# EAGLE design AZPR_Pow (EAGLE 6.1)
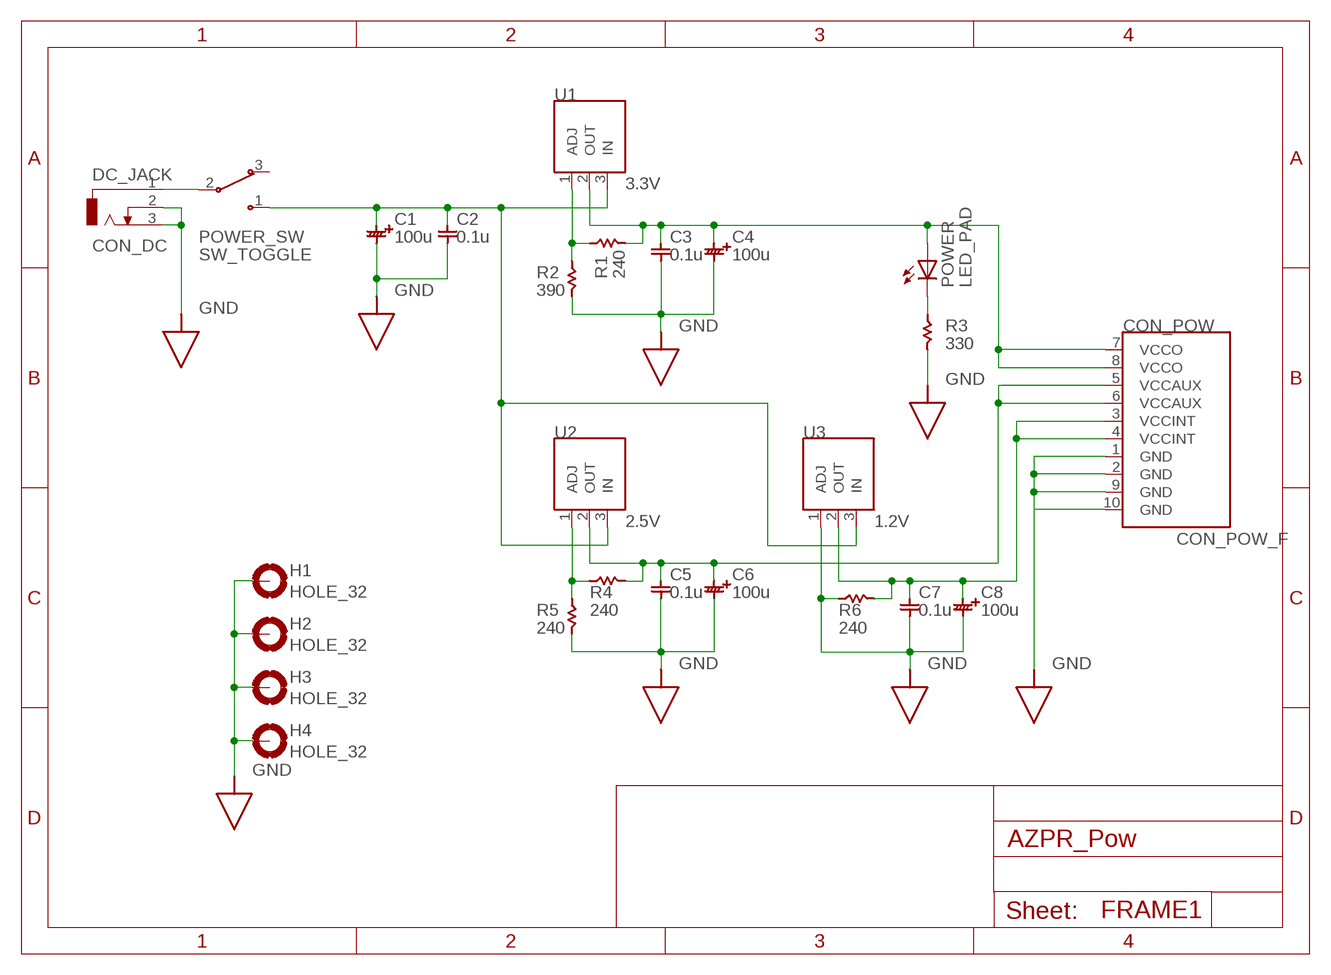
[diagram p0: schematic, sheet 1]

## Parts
C1  100u  CAP_PAD_ELEC  [PAD_CAP_ELEC_POL]
C2  0.1u  CAP_PAD_CERA  [PAD_CAP_CERA]
C3  0.1u  CAP_PAD_CERA  [PAD_CAP_CERA]
C4  100u  CAP_PAD_ELEC  [PAD_CAP_ELEC_POL]
C5  0.1u  CAP_PAD_CERA  [PAD_CAP_CERA]
C6  100u  CAP_PAD_ELEC  [PAD_CAP_ELEC_POL]
C7  0.1u  CAP_PAD_CERA  [PAD_CAP_CERA]
C8  100u  CAP_PAD_ELEC  [PAD_CAP_ELEC_POL]
CON_POW  CON_POW_F  [PAD_POW_F]
DC_JACK  CON_DC  [CON_DC]
H1  HOLE_32  [HOLE_32]
H2  HOLE_32  [HOLE_32]
H3  HOLE_32  [HOLE_32]
H4  HOLE_32  [HOLE_32]
POWER  LED_PAD  [PAD_LED_POL]
POWER_SW  SW_TOGGLE  [PAD_SW_TOGGLE]
R1  240  REG_PAD_04INCH  [PAD_REG_04INCH]
R2  390  REG_PAD_04INCH  [PAD_REG_04INCH]
R3  330  REG_PAD_04INCH  [PAD_REG_04INCH]
R4  240  REG_PAD_04INCH  [PAD_REG_04INCH]
R5  240  REG_PAD_04INCH  [PAD_REG_04INCH]
R6  240  REG_PAD_04INCH  [PAD_REG_04INCH]
U1  3.3V  UNIT_REG_ADJ  [PAD_REG_317]
U2  2.5V  UNIT_REG_ADJ  [PAD_REG_317]
U3  1.2V  UNIT_REG_ADJ  [PAD_REG_317]

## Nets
GND: C1.2 C2.2 C3.2 C4.2 C5.2 C6.2 C7.2 C8.2 CON_POW.1(GND) CON_POW.2(GND) CON_POW.9(GND) CON_POW.10(GND) DC_JACK.2 DC_JACK.3 H1.B3,2(MOUNT) H2.B3,2(MOUNT) H3.B3,2(MOUNT) H4.B3,2(MOUNT) R2.2 R3.2 R5.2 R6.1 U3.1(ADJ)
N$1: C1.1 C2.1 POWER_SW.1 U1.3(IN) U2.3(IN) U3.3(IN)
N$2: DC_JACK.1 POWER_SW.2
N$3: C7.1 C8.1 CON_POW.3(VCCINT) CON_POW.4(VCCINT) R6.2 U3.2(OUT)
N$4: C3.1 C4.1 CON_POW.7(VCCO) CON_POW.8(VCCO) POWER.A R1.2 U1.2(OUT)
N$7: POWER.C R3.1
N$9: C5.1 C6.1 CON_POW.5(VCCAUX) CON_POW.6(VCCAUX) R4.2 U2.2(OUT)
N$11: R1.1 R2.1 U1.1(ADJ)
N$13: R4.1 R5.1 U2.1(ADJ)
Unconnected: POWER_SW.3

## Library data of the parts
C1 C4 C6 C8 = 00_Respon:CAP_PAD_ELEC: electrolytic capacitorr
C2 C3 C5 C7 = 00_Respon:CAP_PAD_CERA: ceramic capacitor
CON_POW = 00_Respon:CON_POW_F: pin connector - 2*5
DC_JACK = 00_Respon:CON_DC: DC POWER JACK Source: DCJ0202.pdf
H1-H4 = 00_Respon:HOLE_32: Mounting PAD
POWER = 00_Respon:LED_PAD: LED
POWER_SW = 00_Respon:SW_TOGGLE: Toggle Switch PAD package
R1-R6 = 00_Respon:REG_PAD_04INCH: resistor
U1-U3 = 00_Respon:UNIT_REG_ADJ: Regulator LM317 PAD package

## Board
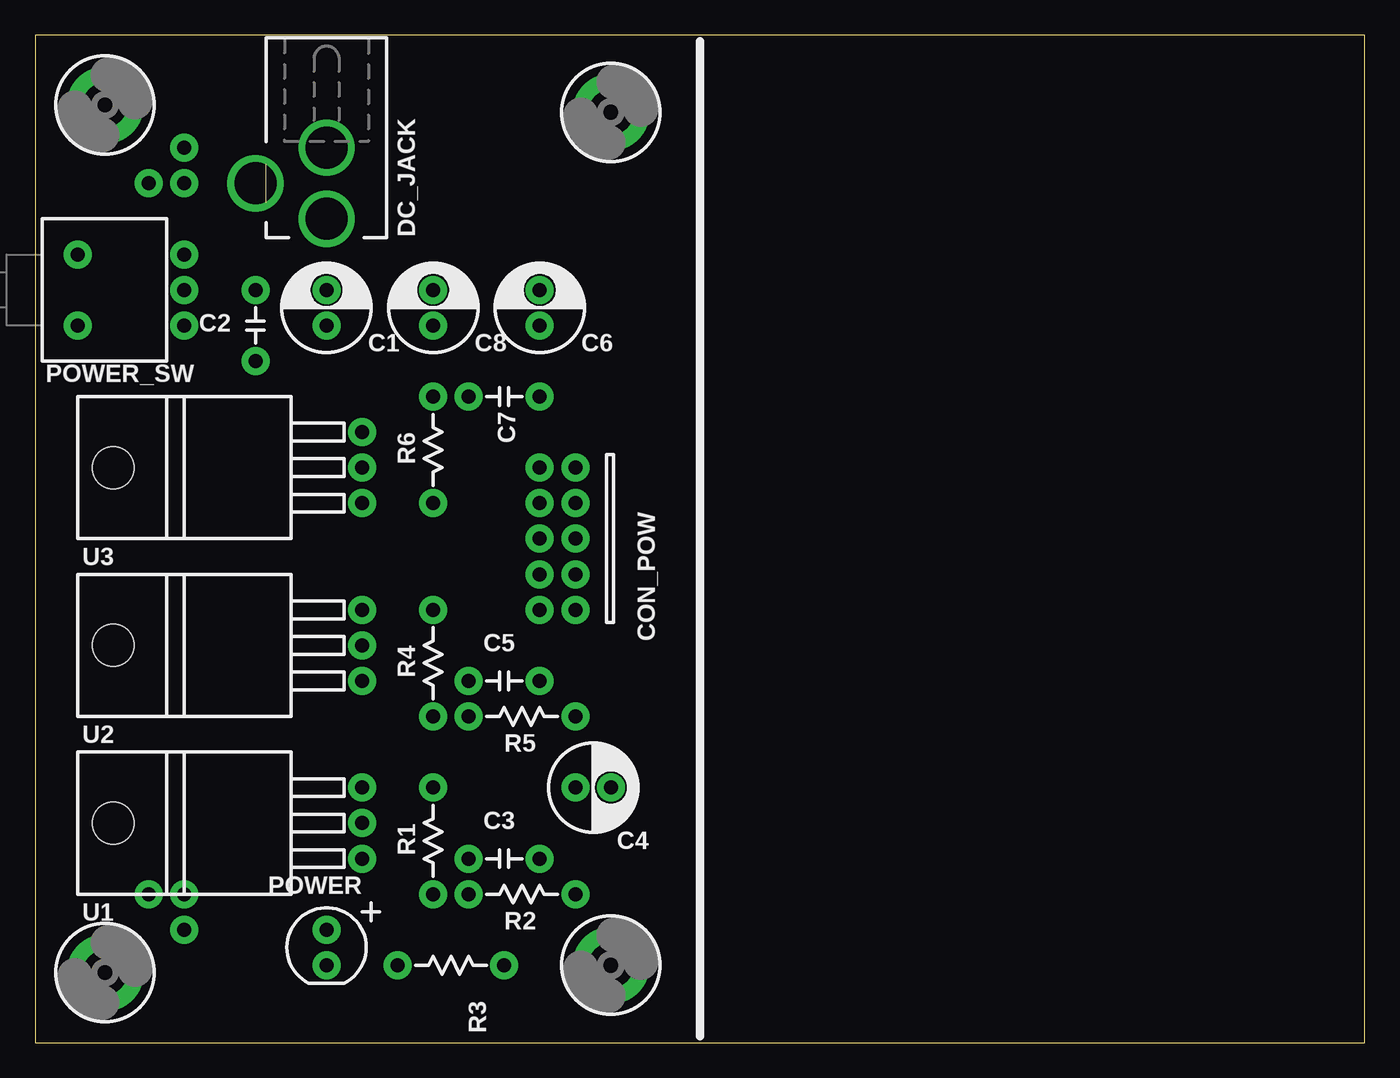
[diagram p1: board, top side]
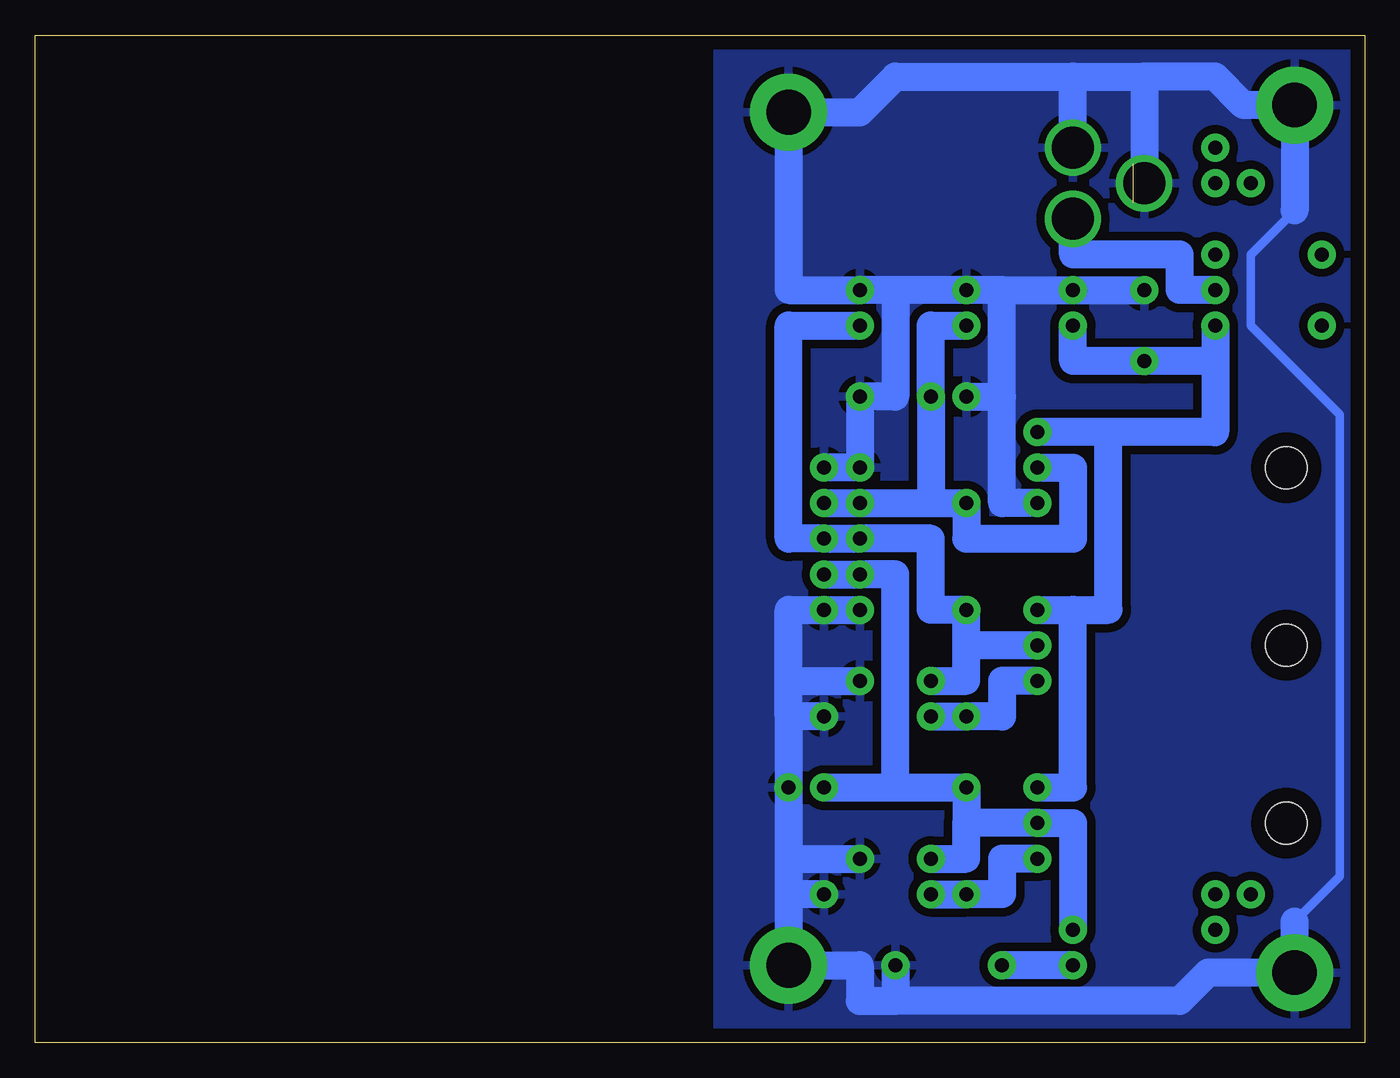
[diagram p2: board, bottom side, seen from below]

Size 95 x 72 mm. Coordinates in mm from the lower left corner, seen from the top.
Outline: 0,0 95,0 95,72 0,72 0,0
Copper layers (1*16): Top 0.035mm / dielectric 1.5mm / Bottom 0.035mm
Design rules: minimum track width 10mil, minimum drill 24mil, track to track 8mil, track to pad 8mil, pad to pad 8mil, via to via 8mil, smd to smd 8mil, copper to edge 40mil, drill to drill 8mil, minimum pad ring 10mil, minimum via ring 8mil, stop-mask expansion 4mil, vias tented up to drill 0mil, thermal gap 20mil

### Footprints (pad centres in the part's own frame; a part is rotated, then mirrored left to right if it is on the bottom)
PAD_CAP_ELEC_POL = drill 1 pad 2: 1 0,2.54; 2 0,0
PAD_CAP_CERA = drill 1 pad 2: 1 0,0; 2 0,5.08
PAD_POW_F = drill 1 pad 2: 1 -1.27,5.08; 2 1.27,5.08; 3 -1.27,2.54; 4 1.27,2.54; 5 -1.27,0; 6 1.27,0; 7 -1.27,-2.54; 8 1.27,-2.54; 9 -1.27,-5.08; 10 1.27,-5.08
CON_DC = drill 3 pad 4: 1 0,2.54; 2 5.08,0; 3 0,-2.54
HOLE_32 = drill 3.2 pad 5.5: B3,2 0,0
PAD_LED_POL = drill 1 pad 2: A 0,0; C 0,2.54
PAD_SW_TOGGLE = drill 1 pad 2: 1 -2.54,0; 2 0,0; 3 2.54,0; 4 -2.54,7.62; 5 2.54,7.62
PAD_REG_04INCH = drill 1 pad 2: 1 0,0; 2 0,7.62
PAD_REG_317 = drill 1 pad 2: 1 -2.54,0; 2 0,0; 3 2.54,0 | hole 3: 0,17.78

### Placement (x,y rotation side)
C1  20.83,53.78 180 top
C2  15.75,48.7 0 top
C3  30.99,13.14 270 top
C4  41.15,18.22 90 top
C5  30.99,25.84 270 top
C6  36.07,53.78 180 top
C7  30.99,46.16 270 top
C8  28.45,53.78 180 top
CON_POW  37.34,36 0 top
DC_JACK  20.83,61.4 180 top
H1  41.15,66.48 0 top
H2  5,67 0 top
H3  41.15,5.52 0 top
H4  5,5 0 top
POWER  20.83,8.06 180 top
POWER_SW  10.67,53.78 90 top
R1  28.45,10.6 0 top
R2  30.99,10.6 270 top
R3  25.91,5.52 270 top
R4  28.45,23.3 0 top
R5  30.99,23.3 270 top
R6  28.45,46.16 180 top
U1  23.37,15.68 90 top
U2  23.37,28.38 90 top
U3  23.37,41.08 90 top

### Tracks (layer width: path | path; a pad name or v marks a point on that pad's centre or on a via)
GND
  Bottom 0.6: 5,8.65 1.78,11.87 1.78,44.89 8.13,51.24 8.13,56.32 5,59.45
  Bottom 2: U3.1 25.91,38.54 25.91,46.16 | 25.91,46.16 25.91,53.78 | 25.91,53.78 C1.2 C2.2 | 25.91,53.78 C8.2 33.53,53.78 | 33.53,53.78 C6.2 41.15,53.78 H1.B3,2 36.07,66.48 33.53,69.02 20.83,69.02 | R6.1 25.91,46.16 | 33.53,53.78 33.53,46.16 C7.2 CON_POW.1 CON_POW.2 | CON_POW.9 CON_POW.10 41.15,30.92 41.15,25.84 | R5.2 41.15,23.3 | 41.15,23.3 C4.2 41.15,13.14 | 41.15,13.14 C3.2 | 41.15,13.14 41.15,10.6 | 41.15,10.6 H3.B3,2 36.07,5.52 36.07,2.98 33.53,2.98 | R2.2 41.15,10.6 | R3.2 33.53,2.98 | 33.53,2.98 13.21,2.98 11.19,5 H4.B3,2 5,8.65 | 20.83,69.02 15.75,69.02 | 15.75,69.02 DC_JACK.2 | DC_JACK.3 20.83,69.02 | 15.75,69.02 10.67,69.02 8.65,67 H2.B3,2 5,59.45 | 41.15,23.3 41.15,25.84 | 41.15,25.84 C5.2
  pour Bottom (isolate 0.6): 0.51,71.56 46.23,71.56 46.23,0.44 0.51,0.44
N$1
  Bottom 2: POWER_SW.1 10.67,48.7 | 10.67,48.7 10.67,43.62 18.29,43.62 | 18.29,43.62 U3.3 | 10.67,48.7 C2.1 20.83,48.7 C1.1 | U2.3 20.83,30.92 | 20.83,30.92 18.29,30.92 18.29,43.62 | U1.3 20.83,18.22 20.83,30.92
N$2
  Bottom 2: POWER_SW.2 13.21,53.78 13.21,56.32 20.83,56.32 DC_JACK.1
N$3
  Bottom 2: CON_POW.4 CON_POW.3 30.99,38.54 | U3.2 20.83,41.08 20.83,36 28.45,36 R6.2 30.99,38.54 | 30.99,38.54 C7.1 30.99,51.24 C8.1
N$4
  Bottom 2: CON_POW.8 CON_POW.7 33.53,33.46 33.53,18.22 | 28.45,15.68 R1.2 33.53,18.22 | 28.45,15.68 28.45,13.14 C3.1 | POWER.A 20.83,15.68 U1.2 28.45,15.68 | C4.1 33.53,18.22
N$5  (via drill 1 pad 2)
  other vias: 10.67,61.4
N$6  (via drill 1 pad 2)
  other vias: 10.67,63.94
N$7
  Bottom 2: POWER.C R3.1
N$8  (via drill 1 pad 2)
  other vias: 8.13,61.4
N$9
  Bottom 2: C6.1 41.15,51.24 41.15,36 CON_POW.6 CON_POW.5 30.99,36 30.99,30.92 R4.2 28.45,28.38 | U2.2 28.45,28.38 | C5.1 28.45,25.84 28.45,28.38
N$10  (via drill 1 pad 2)
  other vias: 8.13,10.6
N$11
  Bottom 2: U1.1 25.91,13.14 25.91,10.6 R1.1 R2.1
N$13
  Bottom 2: R5.1 R4.1 25.91,23.3 25.91,25.84 U2.1
N$14  (via drill 1 pad 2)
  other vias: 10.67,10.6
N$15  (via drill 1 pad 2)
  other vias: 10.67,8.06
